VAR_GLOBAL
//***********************************************
//!!!!!以下对应实际硬件，绝对禁止在程序中使用!!!!
//***********************************************
	GB_EL1889 	AT %I*: ARRAY[1..3, 0..15] OF BOOL;
	GB_EL3164 	AT %I*: ARRAY[1..4, 1..4]  OF INT;
	GB_EL3124 	AT %I*: ARRAY[1..1, 1..4]  OF INT;
	GB_EL6022 	AT %Q*: ARRAY[1..1, 0..21] OF USINT;
	GB_EL2889 	AT %Q*: ARRAY[1..1, 0..15] OF BOOL;
	GB_EV		AT %Q*:	ARRAY[1..5] OF dut_EX260_SEC;
	
	EXH_EL1889  AT %I*: ARRAY[1..5, 0..15] OF BOOL;
	EXH_EL3124  AT %I*: ARRAY[1..5, 1..4]  OF INT;
	EXH_EL3164  AT %I*: ARRAY[1..4, 1..4]  OF INT;
	EXH_EL2889  AT %Q*: ARRAY[1..1, 0..15] OF BOOL;
	EXH_EV		AT %Q*:	ARRAY[1..1] OF dut_EX260_SEC;
	
	OP_EL1889   AT %I*: ARRAY[1..1, 0..15] OF BOOL;
	OP_EL3124   AT %I*: ARRAY[1..2, 1..4]  OF INT;
	
//***********************************************
//!!!!!以下对对应软件，允许在程序中使用
//***********************************************
	//程序内部使用输入
	stGBI			:	dut_GB_Input;
	stEXHI			:	dut_EXH_Input;
	stOPI			:	dut_OP_INPUT;
	
	//程序内部使用输出
	stGBQ			:	dut_GB_Output;
	stEXHQ			:	dut_EXH_Output;
	stOPQ			:	dut_OP_Output;
	
	
	stILK			:	dut_Interlock ;
	aILK_AV			:	ARRAY[1..250] OF BOOL ;
	aVAC			:	ARRAY[1..10]  OF BOOL ;
	
	aAV				:	ARRAY[1..250] OF BOOL ;
	bAV540			: 	BOOL;
	
END_VAR
